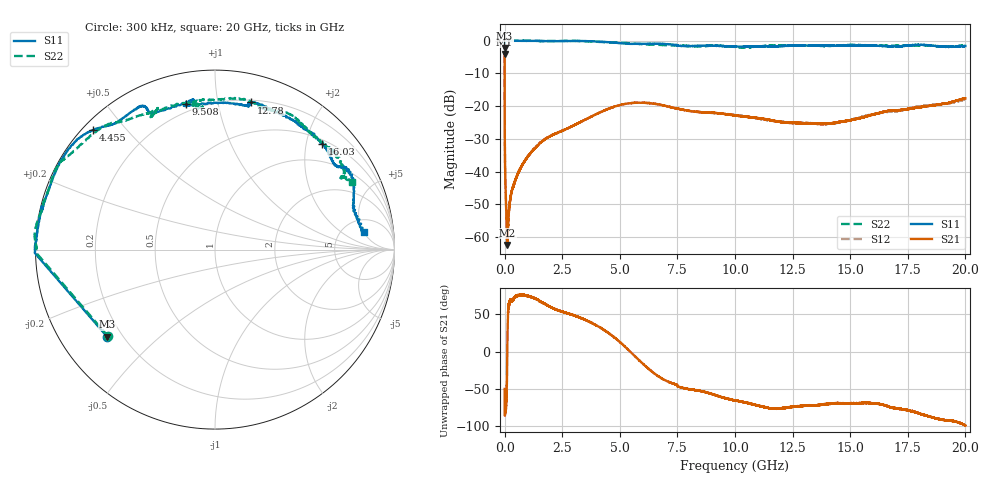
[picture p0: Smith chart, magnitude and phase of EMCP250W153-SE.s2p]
!EMCP250W153
!Johanson Technology Inc.
!www.johansontechnology.com
!Test Board Conditions:
!Substrate Type  RO4350B
!Substrate Thickness  10 mil
!Substrate Dk  3.66
!TL Type: GCPW
!TL Trace Width  20 mil
!TL Gap  10 mil
!PART MODE SINGLE ENDED (AKA BYPASS)
!DUT TOPOLOGY	SERIES-SHUNT
# MHz S  dB  R 50
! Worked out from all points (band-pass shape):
!   20001 points, 300 kHz to 20 GHz, reference 50 ohm
!   highest |S21| = -4.07 dB at 300 kHz (marker M1); lowest = -62.3 dB at 115.3 MHz (marker M2)
!   |S21| within 3 dB of the highest: start of sweep to 586.6 kHz
!   lowest |S11| = -2.2 dB at 300 kHz (marker M3), VSWR 7.78, Z = 7.21 - j17.4 ohm
!   |S11| at or under -10 dB: nowhere
!   |S22| runs from -2.3 to 0.1 dB; largest |S21 - S12| = 0.0074
!   S11 on the Smith chart (normalised r, x): 300 kHz: 0.14, -0.35; 4.455 GHz: 0.03, +0.41; 9.508 GHz: 0.15, +0.81; 12.78 GHz: 0.22, +1.25; 16.03 GHz: 0.57, +2.32; 20 GHz: 7.64, +4.97
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0.3  -2.24 -141.0  -4.07 -49.9  -4.04 -50.0  -2.30 -141.0
77.299  0.03 179.6  -53.42 -67.0  -53.67 -69.7  -0.03 179.7
115.298  0.03 179.3  -62.35 -1.4  -62.75 -1.3  -0.04 179.4
173.297  0.02 178.8  -52.82 60.3  -53.34 58.3  -0.03 179.0
295.296  0.01 177.9  -46.29 67.9  -46.33 68.8  -0.01 178.2
499.293  -0.02 176.0  -41.86 73.1  -41.86 74.1  0.04 177.0
1088.284  -0.06 170.4  -34.58 73.5  -34.63 73.7  0.03 171.8
1836.272  -0.11 164.7  -29.73 61.8  -29.64 62.0  -0.12 161.1
3334.25  -0.09 146.1  -24.67 44.3  -24.69 44.4  -0.11 150.0
4455.233  -0.43 135.5  -20.95 25.8  -20.94 25.7  -0.48 141.5
6667.2  -0.91 117.3  -19.46 -33.0  -19.40 -33.3  -1.28 121.6
7600.186  -1.57 113.5  -20.89 -47.4  -20.89 -47.2  -1.44 112.2
8624.171  -1.48 98.9  -21.88 -53.6  -21.87 -53.9  -1.67 114.7
9508.157  -1.62 101.4  -22.34 -61.7  -22.32 -60.8  -1.60 100.1
10000.15  -1.76 101.5  -22.81 -65.3  -22.68 -65.1  -1.89 95.3
11439.13  -1.71 78.4  -24.09 -75.0  -24.27 -74.8  -1.59 97.1
12784.11  -1.47 76.1  -25.17 -73.2  -25.06 -73.0  -1.44 83.0
13334.1  -1.50 71.4  -25.22 -71.8  -25.20 -72.4  -1.45 75.9
16034.06  -1.50 44.6  -22.49 -69.3  -22.42 -70.5  -1.42 54.7
16667.05  -1.74 37.0  -21.39 -73.4  -21.66 -73.7  -1.51 50.9
18026.03  -1.31 29.1  -20.32 -82.9  -20.17 -82.4  -1.41 35.3
20000  -1.60 6.9  -17.62 -98.6  -17.94 -96.5  -1.36 26.0
